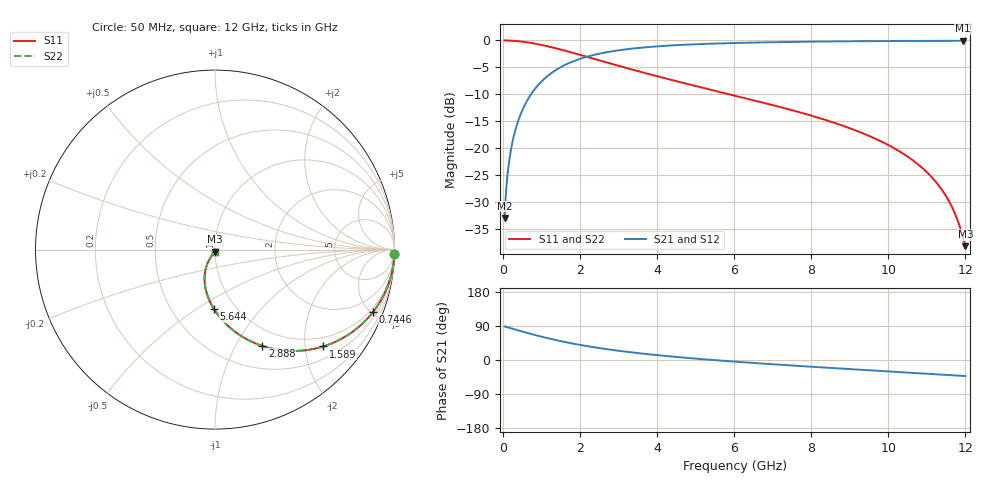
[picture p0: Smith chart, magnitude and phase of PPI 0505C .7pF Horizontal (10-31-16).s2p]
# MHz S MA R 50
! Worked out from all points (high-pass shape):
!   1601 points, 50 MHz to 12 GHz, reference 50 ohm
!   highest |S21| = -0.07 dB at 11.93 GHz (marker M1); lowest = -32.9 dB at 50 MHz (marker M2)
!   |S21| within 3 dB of the highest: 2.159 GHz to end of sweep
!   lowest |S11| = -38.1 dB at 12 GHz (marker M3), VSWR 1.03, Z = 49.8 - j1.23 ohm
!   |S11| at or under -10 dB: 5.895 GHz to end of sweep
!   |S22| runs from -38.1 to 0.0 dB; largest |S21 - S12| = 0
!   S11 on the Smith chart (normalised r, x): 50 MHz: 1, -77; 744.6 MHz: 0.77, -5.16; 1.589 GHz: 0.77, -2.40; 2.888 GHz: 0.77, -1.29; 5.644 GHz: 0.79, -0.59; 12 GHz: 1.00, -0.02
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50  0.9997 -1.5  0.02268 88.5  0.02268 88.5  0.9997 -1.5
169.5  0.997 -5.0  0.0767 85.0  0.0767 85.0  0.997 -5.0
221.7812  0.9949 -6.6  0.1001 83.4  0.1001 83.4  0.9949 -6.6
289  0.9915 -8.6  0.1301 81.4  0.1301 81.4  0.9915 -8.6
483.1875  0.9767 -14.2  0.2143 75.8  0.2143 75.8  0.9767 -14.2
744.5938  0.947 -21.5  0.3203 68.5  0.3203 68.5  0.947 -21.5
1118.031  0.8909 -31.1  0.4531 58.8  0.4531 58.8  0.8909 -31.1
1588.562  0.809 -41.9  0.5862 48.0  0.5862 48.0  0.809 -41.9
2044.156  0.7292 -50.7  0.6823 39.2  0.6823 39.2  0.7292 -50.7
2888.125  0.5982 -63.8  0.7986 25.9  0.7986 25.9  0.5982 -63.8
4038.312  0.4628 -77.1  0.883 12.5  0.883 12.5  0.4628 -77.1
5644.094  0.3326 -90.8  0.9388 -1.5  0.9388 -1.5  0.3326 -90.8
6025  0.3081 -93.6  0.9469 -4.4  0.9469 -4.4  0.3081 -93.6
8019.156  0.2002 -106.4  0.9742 -17.9  0.9742 -17.9  0.2002 -106.4
9139.469  0.1473 -112.7  0.983 -24.8  0.983 -24.8  0.1473 -112.7
10013.31  0.1067 -116.9  0.9877 -30.2  0.9877 -30.2  0.1067 -116.9
10715.38  0.07375 -119.4  0.9902 -34.5  0.9902 -34.5  0.07375 -119.4
11245.66  0.04833 -119.6  0.9914 -37.7  0.9914 -37.7  0.04833 -119.6
11641.5  0.0291 -116.2  0.9919 -40.1  0.9919 -40.1  0.0291 -116.2
11790.88  0.02191 -112.1  0.992 -41.0  0.992 -41.0  0.02191 -112.1
11925.31  0.01564 -104.5  0.992 -41.9  0.992 -41.9  0.01564 -104.5
12000  0.0124 -96.6  0.992 -42.3  0.992 -42.3  0.0124 -96.6
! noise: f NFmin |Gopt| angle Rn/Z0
50  0.001452  0.9778  1.292  0.01491
1372  0.005849  0.775  8.288  0.005285
2701  0.009139  0.7191  12.7  0.006363
4031  0.01206  0.6877  17.21  0.007342
5360  0.01481  0.6676  21.72  0.008264
6682  0.01748  0.6546  26.16  0.00917
8012  0.02016  0.6468  30.54  0.0101
9341  0.02289  0.643  34.81  0.01109
1.067e+04  0.02571  0.6428  38.96  0.01217
1.2e+04  0.02867  0.6455  42.98  0.01336
